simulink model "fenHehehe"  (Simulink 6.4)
settings: Solver=ode45  StartTime=0.0  StopTime=500  RelTol=1e-3
libraries: rtsrcs x1, rtsinks x1, simulink x1

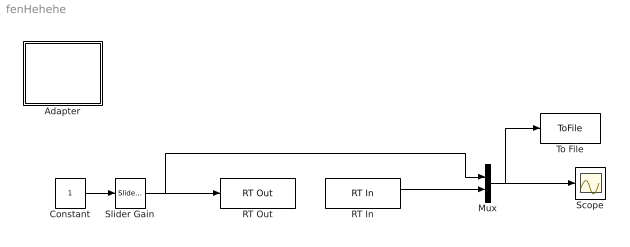
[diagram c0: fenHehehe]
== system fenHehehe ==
  Adapter : Subsystem
  Constant : Constant  Value=1  OutDataType=sfix(16)  ConRadixGroup=Use specified scaling  OutScaling=2^0  SampleTime=inf  FramePeriod=inf
  Mux : Mux  Inputs=2
  RT In : rtsrcs/RT In  Ts=0.5  maxlost=10000  adapter='Adapter'  channels=1
  RT Out : rtsinks/RT Out  Ts=0.5  maxlost=10000  adapter='Adapter'  channels=1
  Scope : Scope
  Slider Gain : simulink/Math Operations/Slider Gain  SystemSampleTime=-1  low=-1  gain=-0.3  high=1
  To File : ToFile  Filename=vystup.mat
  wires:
  Constant/1 -> Slider Gain/1
  Slider Gain/1 -> RT Out/1, Mux/1
  RT In/1 -> Mux/2
  Mux/1 -> To File/1, Scope/1

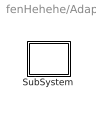
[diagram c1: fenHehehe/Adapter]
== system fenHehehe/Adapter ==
  SubSystem : Subsystem

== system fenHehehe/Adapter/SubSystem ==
